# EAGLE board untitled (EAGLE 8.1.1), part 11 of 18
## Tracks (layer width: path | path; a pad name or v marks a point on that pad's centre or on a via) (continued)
S$10909 (continued)
  Bottom 0: 84.24,134.12 84.26,134.19
S$10910
  Bottom 0: 84.26,134.19 84.28,134.25
S$10911
  Bottom 0: 84.28,134.25 84.28,134.32
S$10912
  Bottom 0: 84.28,134.32 84.28,148.03
S$10913
  Bottom 0: 84.28,148.03 84.28,148.11
S$10914
  Bottom 0: 84.28,148.11 84.26,148.17
S$10915
  Bottom 0: 84.26,148.17 84.24,148.23
S$10916
  Bottom 0: 84.24,148.23 84.2,148.29
S$10917
  Bottom 0: 84.2,148.29 84.16,148.35
S$10918
  Bottom 0: 84.16,148.35 75.22,157.29
S$10919
  Bottom 0: 75.22,157.29 75.16,157.33
S$10920
  Bottom 0: 75.16,157.33 75.1,157.37
S$10921
  Bottom 0: 75.1,157.37 75.04,157.39
S$10922
  Bottom 0: 75.04,157.39 74.97,157.41
S$10923
  Bottom 0: 74.97,157.41 74.9,157.41
S$10924
  Bottom 0: 74.9,157.41 63.82,157.41
S$10925
  Bottom 0: 63.82,157.41 64.06,157.65
S$10926
  Bottom 0: 64.06,157.65 64.16,157.61
S$10927
  Bottom 0: 64.16,157.61 64.46,157.59
S$10928
  Bottom 0: 64.46,157.59 64.76,157.66
S$10929
  Bottom 0: 64.76,157.66 65.02,157.81
S$10930
  Bottom 0: 65.02,157.81 65.22,158.03
S$10931
  Bottom 0: 65.22,158.03 65.36,158.3
S$10932
  Bottom 0: 65.36,158.3 65.41,158.6
S$10933
  Bottom 0: 65.41,158.6 65.36,158.9
S$10934
  Bottom 0: 65.36,158.9 65.22,159.18
S$10935
  Bottom 0: 65.22,159.18 65.02,159.4
S$10936
  Bottom 0: 65.02,159.4 64.76,159.55
S$10937
  Bottom 0: 64.76,159.55 64.46,159.61
S$10938
  Bottom 0: 64.46,159.61 64.16,159.59
S$10939
  Bottom 0: 64.16,159.59 63.88,159.48
S$10940
  Bottom 0: 63.88,159.48 63.64,159.29
S$10941
  Bottom 0: 63.64,159.29 63.47,159.04
S$10942
  Bottom 0: 63.47,159.04 63.38,158.75
S$10943
  Bottom 0: 63.38,158.75 63.38,158.45
S$10944
  Bottom 0: 63.38,158.45 63.44,158.28
S$10945
  Bottom 0: 63.44,158.28 63.34,158.18
S$10946
  Bottom 0: 63.34,158.18 59.58,158.18
S$10947
  Bottom 0: 59.58,158.18 67.09,165.69
S$10948
  Bottom 0: 67.09,165.69 67.02,165.43
S$10949
  Bottom 0: 67.02,165.43 67.02,165.11
S$10950
  Bottom 0: 67.02,165.11 67.11,164.79
S$10951
  Bottom 0: 67.11,164.79 67.28,164.52
S$10952
  Bottom 0: 67.28,164.52 67.51,164.3
S$10953
  Bottom 0: 67.51,164.3 67.8,164.15
S$10954
  Bottom 0: 67.8,164.15 68.12,164.08
S$10955
  Bottom 0: 68.12,164.08 68.45,164.1
S$10956
  Bottom 0: 68.45,164.1 68.75,164.21
S$10957
  Bottom 0: 68.75,164.21 69.02,164.4
S$10958
  Bottom 0: 69.02,164.4 69.22,164.65
S$10959
  Bottom 0: 69.22,164.65 69.35,164.95
S$10960
  Bottom 0: 69.35,164.95 69.37,165.07
S$10961
  Bottom 0: 69.37,165.07 73.78,165.07
S$10962
  Bottom 0: 73.78,165.07 73.69,164.84
S$10963
  Bottom 0: 73.69,164.84 73.69,164.58
S$10964
  Bottom 0: 73.69,164.58 73.78,164.35
S$10965
  Bottom 0: 73.78,164.35 73.92,164.2
S$10966
  Bottom 0: 73.92,164.2 73.92,162.77
S$10967
  Bottom 0: 73.92,162.77 73.92,162.7
S$10968
  Bottom 0: 73.92,162.7 73.94,162.63
S$10969
  Bottom 0: 73.94,162.63 73.97,162.57
S$10970
  Bottom 0: 73.97,162.57 74,162.51
S$10971
  Bottom 0: 74,162.51 74.05,162.46
S$10972
  Bottom 0: 74.05,162.46 84.67,151.83
S$10973
  Bottom 0: 84.67,151.83 84.67,131.08
S$10974
  Bottom 0: 84.67,131.08 76.56,122.97
S$10975
  Bottom 0: 76.56,122.97 76.52,122.92
S$10976
  Bottom 0: 76.52,122.92 76.48,122.86
S$10977
  Bottom 0: 76.48,122.86 76.45,122.8
S$10978
  Bottom 0: 76.45,122.8 76.44,122.73
S$10979
  Bottom 0: 76.44,122.73 76.43,122.66
S$10980
  Bottom 0: 76.43,122.66 76.43,116.28
S$10981
  Bottom 0: 76.43,116.28 76.42,116.3
S$10982
  Bottom 0: 76.42,116.3 76.38,116.38
S$10983
  Bottom 0: 76.38,116.38 76.32,116.44
S$10984
  Bottom 0: 76.32,116.44 71.52,121.24
S$10985
  Bottom 0: 71.52,121.24 71.56,121.54
S$10986
  Bottom 0: 71.56,121.54 71.51,121.86
S$10987
  Bottom 0: 71.51,121.86 71.38,122.16
S$10988
  Bottom 0: 71.38,122.16 71.16,122.4
S$10989
  Bottom 0: 71.16,122.4 70.89,122.58
S$10990
  Bottom 0: 70.89,122.58 70.58,122.67
S$10991
  Bottom 0: 70.58,122.67 70.26,122.67
S$10992
  Bottom 0: 70.26,122.67 69.95,122.58
S$10993
  Bottom 0: 69.95,122.58 69.67,122.4
S$10994
  Bottom 0: 69.67,122.4 69.58,122.3
S$10995
  Bottom 0: 69.58,122.3 69.58,122.88
S$10996
  Bottom 0: 69.58,122.88 69.57,122.95
S$10997
  Bottom 0: 69.57,122.95 69.56,123.02
S$10998
  Bottom 0: 69.56,123.02 69.53,123.08
S$10999
  Bottom 0: 69.53,123.08 69.49,123.14
S$11000
  Bottom 0: 69.49,123.14 69.45,123.19
S$11001
  Bottom 0: 69.45,123.19 65.97,126.68
S$11002
  Bottom 0: 65.97,126.68 65.91,126.72
S$11003
  Bottom 0: 65.91,126.72 65.85,126.76
S$11004
  Bottom 0: 65.85,126.76 65.79,126.79
S$11005
  Bottom 0: 65.79,126.79 65.72,126.8
S$11006
  Bottom 0: 65.72,126.8 65.65,126.81
S$11007
  Bottom 0: 65.65,126.81 51.18,126.81
S$11008
  Bottom 0: 51.18,126.81 45.63,132.35
S$11009
  Bottom 0: 45.63,132.35 45.73,132.62
S$11010
  Bottom 0: 45.73,132.62 45.78,132.97
S$11011
  Bottom 0: 45.78,132.97 45.73,133.31
S$11012
  Bottom 0: 45.73,133.31 45.61,133.64
S$11013
  Bottom 0: 45.61,133.64 45.4,133.92
S$11014
  Bottom 0: 45.4,133.92 45.13,134.15
S$11015
  Bottom 0: 45.13,134.15 44.82,134.3
S$11016
  Bottom 0: 44.82,134.3 44.47,134.36
S$11017
  Bottom 0: 44.47,134.36 44.12,134.34
S$11018
  Bottom 0: 44.12,134.34 43.79,134.23
S$11019
  Bottom 0: 43.79,134.23 43.49,134.05
S$11020
  Bottom 0: 43.49,134.05 43.25,133.79
S$11021
  Bottom 0: 43.25,133.79 43.08,133.48
S$11022
  Bottom 0: 43.08,133.48 42.99,133.14
S$11023
  Bottom 0: 42.99,133.14 42.99,132.79
S$11024
  Bottom 0: 42.99,132.79 43.08,132.46
S$11025
  Bottom 0: 43.08,132.46 43.25,132.15
S$11026
  Bottom 0: 43.25,132.15 43.49,131.89
S$11027
  Bottom 0: 43.49,131.89 43.79,131.7
S$11028
  Bottom 0: 43.79,131.7 44.12,131.6
S$11029
  Bottom 0: 44.12,131.6 44.47,131.58
S$11030
  Bottom 0: 44.47,131.58 44.82,131.64
S$11031
  Bottom 0: 44.82,131.64 45,131.73
S$11032
  Bottom 0: 45,131.73 50.68,126.05
S$11033
  Bottom 0: 50.68,126.05 50.73,126.01
S$11034
  Bottom 0: 50.73,126.01 50.8,125.97
S$11035
  Bottom 0: 50.8,125.97 50.86,125.94
S$11036
  Bottom 0: 50.86,125.94 50.92,125.93
S$11037
  Bottom 0: 50.92,125.93 50.99,125.92
S$11038
  Bottom 0: 50.99,125.92 53.56,125.92
S$11039
  Bottom 0: 53.56,125.92 53.51,125.91
S$11040
  Bottom 0: 53.51,125.91 53.22,125.77
S$11041
  Bottom 0: 53.22,125.77 52.99,125.54
S$11042
  Bottom 0: 52.99,125.54 52.82,125.27
S$11043
  Bottom 0: 52.82,125.27 52.73,124.95
S$11044
  Bottom 0: 52.73,124.95 52.73,124.63
S$11045
  Bottom 0: 52.73,124.63 52.82,124.31
S$11046
  Bottom 0: 52.82,124.31 52.99,124.04
S$11047
  Bottom 0: 52.99,124.04 53.22,123.81
S$11048
  Bottom 0: 53.22,123.81 53.51,123.67
S$11049
  Bottom 0: 53.51,123.67 53.83,123.6
S$11050
  Bottom 0: 53.83,123.6 54.16,123.62
S$11051
  Bottom 0: 54.16,123.62 54.25,123.65
S$11052
  Bottom 0: 54.25,123.65 57.6,120.3
S$11053
  Bottom 0: 57.6,120.3 57.6,108.63
S$11054
  Bottom 0: 57.6,108.63 57.6,108.54
S$11055
  Bottom 0: 57.6,108.54 57.63,108.45
S$11056
  Bottom 0: 57.63,108.45 57.66,108.37
S$11057
  Bottom 0: 57.66,108.37 57.71,108.3
S$11058
  Bottom 0: 57.71,108.3 57.77,108.23
S$11059
  Bottom 0: 57.77,108.23 59.92,106.08
S$11060
  Bottom 0: 59.92,106.08 59.88,105.9
S$11061
  Bottom 0: 59.88,105.9 59.88,105.58
S$11062
  Bottom 0: 59.88,105.58 59.96,105.26
S$11063
  Bottom 0: 59.96,105.26 60.14,104.99
S$11064
  Bottom 0: 60.14,104.99 60.37,104.77
S$11065
  Bottom 0: 60.37,104.77 60.49,104.7
S$11066
  Bottom 0: 60.49,104.7 60.49,103.2
S$11067
  Bottom 0: 60.49,103.2 59.64,102.36
S$11068
  Bottom 0: 47.94,120.4 49.72,120.4
S$11069
  Bottom 0: 49.72,120.4 49.79,120.41
S$11070
  Bottom 0: 49.79,120.41 49.87,120.45
S$11071
  Bottom 0: 49.87,120.45 49.92,120.5
S$11072
  Bottom 0: 49.92,120.5 49.96,120.57
S$11073
  Bottom 0: 49.96,120.57 49.97,120.65
S$11074
  Bottom 0: 49.97,120.65 49.97,122.43
S$11075
  Bottom 0: 49.97,122.43 49.96,122.5
S$11076
  Bottom 0: 49.96,122.5 49.92,122.58
S$11077
  Bottom 0: 49.92,122.58 49.87,122.63
S$11078
  Bottom 0: 49.87,122.63 49.79,122.67
S$11079
  Bottom 0: 49.79,122.67 49.72,122.68
S$11080
  Bottom 0: 49.72,122.68 49.27,122.68
S$11081
  Bottom 0: 49.27,122.68 49.27,122.81
S$11082
  Bottom 0: 49.27,122.81 49.21,123.03
S$11083
  Bottom 0: 49.21,123.03 49.05,123.19
S$11084
  Bottom 0: 49.05,123.19 48.83,123.25
S$11085
  Bottom 0: 48.83,123.25 48.46,123.25
S$11086
  Bottom 0: 48.46,123.25 47.38,124.33
S$11087
  Bottom 0: 47.38,124.33 47.44,124.47
S$11088
  Bottom 0: 47.44,124.47 47.49,124.79
S$11089
  Bottom 0: 47.49,124.79 47.44,125.11
S$11090
  Bottom 0: 47.44,125.11 47.31,125.41
S$11091
  Bottom 0: 47.31,125.41 47.11,125.66
S$11092
  Bottom 0: 47.11,125.66 46.84,125.85
S$11093
  Bottom 0: 46.84,125.85 46.54,125.96
S$11094
  Bottom 0: 46.54,125.96 46.21,125.98
S$11095
  Bottom 0: 46.21,125.98 45.89,125.91
S$11096
  Bottom 0: 45.89,125.91 45.6,125.77
S$11097
  Bottom 0: 45.6,125.77 45.37,125.54
S$11098
  Bottom 0: 45.37,125.54 45.2,125.27
S$11099
  Bottom 0: 45.2,125.27 45.11,124.95
S$11100
  Bottom 0: 45.11,124.95 45.11,124.63
S$11101
  Bottom 0: 45.11,124.63 45.2,124.31
S$11102
  Bottom 0: 45.2,124.31 45.37,124.04
S$11103
  Bottom 0: 45.37,124.04 45.6,123.81
S$11104
  Bottom 0: 45.6,123.81 45.89,123.67
S$11105
  Bottom 0: 45.89,123.67 46.21,123.6
S$11106
  Bottom 0: 46.21,123.6 46.54,123.62
S$11107
  Bottom 0: 46.54,123.62 46.76,123.7
S$11108
  Bottom 0: 46.76,123.7 47.81,122.64
S$11109
  Bottom 0: 47.81,122.64 47.79,122.63
S$11110
  Bottom 0: 47.79,122.63 47.74,122.58
S$11111
  Bottom 0: 47.74,122.58 47.69,122.5
S$11112
  Bottom 0: 47.69,122.5 47.69,122.43
S$11113
  Bottom 0: 47.69,122.43 47.69,120.65
S$11114
  Bottom 0: 47.69,120.65 47.69,120.57
S$11115
  Bottom 0: 47.69,120.57 47.74,120.5
S$11116
  Bottom 0: 47.74,120.5 47.79,120.45
S$11117
  Bottom 0: 47.79,120.45 47.86,120.41
S$11118
  Bottom 0: 47.86,120.41 47.94,120.4
S$11119
  Bottom 0: 57.17,129.04 57.52,129.1
S$11120
  Bottom 0: 57.52,129.1 57.84,129.25
S$11121
  Bottom 0: 57.84,129.25 58.1,129.47
S$11122
  Bottom 0: 58.1,129.47 58.31,129.76
S$11123
  Bottom 0: 58.31,129.76 58.44,130.08
S$11124
  Bottom 0: 58.44,130.08 58.49,130.43
S$11125
  Bottom 0: 58.49,130.43 58.44,130.77
S$11126
  Bottom 0: 58.44,130.77 58.31,131.1
S$11127
  Bottom 0: 58.31,131.1 58.1,131.38
S$11128
  Bottom 0: 58.1,131.38 57.84,131.61
S$11129
  Bottom 0: 57.84,131.61 57.52,131.76
S$11130
  Bottom 0: 57.52,131.76 57.17,131.82
S$11131
  Bottom 0: 57.17,131.82 56.83,131.8
S$11132
  Bottom 0: 56.83,131.8 56.49,131.69
S$11133
  Bottom 0: 56.49,131.69 56.46,131.67
S$11134
  Bottom 0: 56.46,131.67 55.89,132.25
S$11135
  Bottom 0: 55.89,132.25 55.84,132.29
S$11136
  Bottom 0: 55.84,132.29 55.78,132.33
S$11137
  Bottom 0: 55.78,132.33 55.72,132.35
S$11138
  Bottom 0: 55.72,132.35 55.65,132.37
S$11139
  Bottom 0: 55.65,132.37 55.58,132.38
S$11140
  Bottom 0: 55.58,132.38 51.01,132.38
S$11141
  Bottom 0: 51.01,132.38 50.94,132.51
S$11142
  Bottom 0: 50.94,132.51 50.74,132.72
S$11143
  Bottom 0: 50.74,132.72 50.48,132.88
S$11144
  Bottom 0: 50.48,132.88 50.18,132.94
S$11145
  Bottom 0: 50.18,132.94 49.88,132.92
S$11146
  Bottom 0: 49.88,132.92 49.6,132.81
S$11147
  Bottom 0: 49.6,132.81 49.36,132.62
S$11148
  Bottom 0: 49.36,132.62 49.19,132.38
S$11149
  Bottom 0: 49.19,132.38 49.1,132.09
S$11150
  Bottom 0: 49.1,132.09 49.1,131.78
S$11151
  Bottom 0: 49.1,131.78 49.19,131.49
S$11152
  Bottom 0: 49.19,131.49 49.36,131.24
S$11153
  Bottom 0: 49.36,131.24 49.6,131.05
S$11154
  Bottom 0: 49.6,131.05 49.88,130.94
S$11155
  Bottom 0: 49.88,130.94 50.18,130.92
S$11156
  Bottom 0: 50.18,130.92 50.48,130.99
S$11157
  Bottom 0: 50.48,130.99 50.74,131.14
S$11158
  Bottom 0: 50.74,131.14 50.94,131.36
S$11159
  Bottom 0: 50.94,131.36 51.01,131.49
S$11160
  Bottom 0: 51.01,131.49 55.4,131.49
S$11161
  Bottom 0: 55.4,131.49 55.84,131.04
S$11162
  Bottom 0: 55.84,131.04 55.79,130.94
S$11163
  Bottom 0: 55.79,130.94 55.7,130.6
S$11164
  Bottom 0: 55.7,130.6 55.7,130.25
S$11165
  Bottom 0: 55.7,130.25 55.79,129.92
S$11166
  Bottom 0: 55.79,129.92 55.96,129.61
S$11167
  Bottom 0: 55.96,129.61 56.2,129.35
S$11168
  Bottom 0: 56.2,129.35 56.49,129.16
S$11169
  Bottom 0: 56.49,129.16 56.83,129.06
S$11170
  Bottom 0: 56.83,129.06 57.17,129.04
S$11171
  Bottom 0: 83.52,149.97 83.81,150.04
S$11172
  Bottom 0: 83.81,150.04 84.08,150.19
S$11173
  Bottom 0: 84.08,150.19 84.28,150.41
S$11174
  Bottom 0: 84.28,150.41 84.41,150.68
S$11175
  Bottom 0: 84.41,150.68 84.46,150.98
S$11176
  Bottom 0: 84.46,150.98 84.41,151.28
S$11177
  Bottom 0: 84.41,151.28 84.28,151.56
S$11178
  Bottom 0: 84.28,151.56 84.08,151.78
S$11179
  Bottom 0: 84.08,151.78 83.81,151.93
S$11180
  Bottom 0: 83.81,151.93 83.52,151.99
S$11181
  Bottom 0: 83.52,151.99 83.22,151.97
S$11182
  Bottom 0: 83.22,151.97 82.94,151.86
S$11183
  Bottom 0: 82.94,151.86 82.7,151.67
S$11184
  Bottom 0: 82.7,151.67 82.53,151.43
S$11185
  Bottom 0: 82.53,151.43 82.44,151.13
S$11186
  Bottom 0: 82.44,151.13 82.44,150.83
S$11187
  Bottom 0: 82.44,150.83 82.53,150.54
S$11188
  Bottom 0: 82.53,150.54 82.7,150.29
S$11189
  Bottom 0: 82.7,150.29 82.94,150.1
S$11190
  Bottom 0: 82.94,150.1 83.22,149.99
S$11191
  Bottom 0: 83.22,149.99 83.52,149.97
S$11192
  Bottom 0: 71.75,158.5 73.53,158.5
S$11193
  Bottom 0: 73.53,158.5 73.61,158.51
S$11194
  Bottom 0: 73.61,158.51 73.68,158.55
S$11195
  Bottom 0: 73.68,158.55 73.73,158.6
S$11196
  Bottom 0: 73.73,158.6 73.78,158.67
S$11197
  Bottom 0: 73.78,158.67 73.79,158.75
S$11198
  Bottom 0: 73.79,158.75 73.79,160.53
S$11199
  Bottom 0: 73.79,160.53 73.78,160.6
S$11200
  Bottom 0: 73.78,160.6 73.73,160.68
S$11201
  Bottom 0: 73.73,160.68 73.68,160.73
S$11202
  Bottom 0: 73.68,160.73 73.61,160.77
S$11203
  Bottom 0: 73.61,160.77 73.53,160.78
S$11204
  Bottom 0: 73.53,160.78 73.09,160.78
S$11205
  Bottom 0: 73.09,160.78 73.09,160.91
S$11206
  Bottom 0: 73.09,160.91 73.03,161.13
S$11207
  Bottom 0: 73.03,161.13 72.86,161.29
S$11208
  Bottom 0: 72.86,161.29 72.64,161.35
S$11209
  Bottom 0: 72.64,161.35 72.28,161.35
S$11210
  Bottom 0: 72.28,161.35 71.19,162.43
S$11211
  Bottom 0: 71.19,162.43 71.25,162.57
S$11212
  Bottom 0: 71.25,162.57 71.3,162.89
S$11213
  Bottom 0: 71.3,162.89 71.25,163.22
S$11214
  Bottom 0: 71.25,163.22 71.13,163.51
S$11215
  Bottom 0: 71.13,163.51 70.92,163.77
S$11216
  Bottom 0: 70.92,163.77 70.66,163.96
S$11217
  Bottom 0: 70.66,163.96 70.35,164.06
S$11218
  Bottom 0: 70.35,164.06 70.03,164.08
S$11219
  Bottom 0: 70.03,164.08 69.71,164.02
S$11220
  Bottom 0: 69.71,164.02 69.42,163.87
S$11221
  Bottom 0: 69.42,163.87 69.19,163.65
S$11222
  Bottom 0: 69.19,163.65 69.01,163.37
S$11223
  Bottom 0: 69.01,163.37 68.92,163.06
S$11224
  Bottom 0: 68.92,163.06 68.92,162.73
S$11225
  Bottom 0: 68.92,162.73 69.01,162.42
S$11226
  Bottom 0: 69.01,162.42 69.19,162.14
S$11227
  Bottom 0: 69.19,162.14 69.42,161.92
S$11228
  Bottom 0: 69.42,161.92 69.71,161.77
S$11229
  Bottom 0: 69.71,161.77 70.03,161.71
S$11230
  Bottom 0: 70.03,161.71 70.35,161.73
S$11231
  Bottom 0: 70.35,161.73 70.58,161.8
S$11232
  Bottom 0: 70.58,161.8 71.64,160.75
S$11233
  Bottom 0: 71.64,160.75 71.61,160.73
S$11234
  Bottom 0: 71.61,160.73 71.55,160.68
S$11235
  Bottom 0: 71.55,160.68 71.51,160.6
S$11236
  Bottom 0: 71.51,160.6 71.5,160.53
S$11237
  Bottom 0: 71.5,160.53 71.5,158.75
S$11238
  Bottom 0: 71.5,158.75 71.51,158.67
S$11239
  Bottom 0: 71.51,158.67 71.55,158.6
S$11240
  Bottom 0: 71.55,158.6 71.61,158.55
S$11241
  Bottom 0: 71.61,158.55 71.68,158.51
S$11242
  Bottom 0: 71.68,158.51 71.75,158.5
S$11243
  Bottom 0: 75.02,158.51 75.35,158.51
S$11244
  Bottom 0: 75.35,158.51 75.66,158.6
S$11245
  Bottom 0: 75.66,158.6 75.93,158.78
S$11246
  Bottom 0: 75.93,158.78 76.14,159.02
S$11247
  Bottom 0: 76.14,159.02 76.28,159.32
S$11248
  Bottom 0: 76.28,159.32 76.33,159.64
S$11249
  Bottom 0: 76.33,159.64 76.28,159.96
S$11250
  Bottom 0: 76.28,159.96 76.14,160.26
S$11251
  Bottom 0: 76.14,160.26 75.93,160.5
S$11252
  Bottom 0: 75.93,160.5 75.66,160.68
S$11253
  Bottom 0: 75.66,160.68 75.35,160.77
S$11254
  Bottom 0: 75.35,160.77 75.02,160.77
S$11255
  Bottom 0: 75.02,160.77 74.71,160.68
S$11256
  Bottom 0: 74.71,160.68 74.44,160.5
S$11257
  Bottom 0: 74.44,160.5 74.22,160.26
S$11258
  Bottom 0: 74.22,160.26 74.08,159.96
S$11259
  Bottom 0: 74.08,159.96 74.04,159.64
S$11260
  Bottom 0: 74.04,159.64 74.08,159.32
S$11261
  Bottom 0: 74.08,159.32 74.22,159.02
S$11262
  Bottom 0: 74.22,159.02 74.44,158.78
S$11263
  Bottom 0: 74.44,158.78 74.71,158.6
S$11264
  Bottom 0: 74.71,158.6 75.02,158.51
S$11265
  Bottom 0: 226.34,102.45 226.34,102.49
S$11266
  Bottom 0: 226.34,102.49 226.3,102.81
S$11267
  Bottom 0: 226.3,102.81 226.16,103.11
S$11268
  Bottom 0: 226.16,103.11 225.95,103.35
S$11269
  Bottom 0: 225.95,103.35 225.67,103.53
S$11270
  Bottom 0: 225.67,103.53 225.36,103.62
S$11271
  Bottom 0: 225.36,103.62 225.25,103.62
S$11272
  Bottom 0: 225.25,103.62 219.09,109.79
S$11273
  Bottom 0: 219.09,109.79 219.02,109.85
S$11274
  Bottom 0: 219.02,109.85 218.94,109.9
S$11275
  Bottom 0: 218.94,109.9 218.86,109.93
S$11276
  Bottom 0: 218.86,109.93 218.78,109.95
S$11277
  Bottom 0: 218.78,109.95 218.68,109.96
S$11278
  Bottom 0: 218.68,109.96 218.59,109.96
S$11279
  Bottom 0: 218.59,109.96 218.44,110.1
S$11280
  Bottom 0: 218.44,110.1 218.75,110.01
S$11281
  Bottom 0: 218.75,110.01 219.09,109.99
S$11282
  Bottom 0: 219.09,109.99 219.44,110.05
S$11283
  Bottom 0: 219.44,110.05 219.76,110.2
S$11284
  Bottom 0: 219.76,110.2 220.03,110.42
S$11285
  Bottom 0: 220.03,110.42 220.23,110.71
S$11286
  Bottom 0: 220.23,110.71 220.36,111.03
S$11287
  Bottom 0: 220.36,111.03 220.41,111.38
S$11288
  Bottom 0: 220.41,111.38 220.36,111.72
S$11289
  Bottom 0: 220.36,111.72 220.23,112.05
S$11290
  Bottom 0: 220.23,112.05 220.03,112.33
S$11291
  Bottom 0: 220.03,112.33 219.76,112.56
S$11292
  Bottom 0: 219.76,112.56 219.44,112.71
S$11293
  Bottom 0: 219.44,112.71 219.09,112.77
S$11294
  Bottom 0: 219.09,112.77 218.75,112.75
S$11295
  Bottom 0: 218.75,112.75 218.41,112.64
S$11296
  Bottom 0: 218.41,112.64 218.12,112.46
S$11297
  Bottom 0: 218.12,112.46 217.91,112.23
S$11298
  Bottom 0: 217.91,112.23 217.91,115.83
S$11299
  Bottom 0: 217.91,115.83 219.46,117.38
S$11300
  Bottom 0: 219.46,117.38 219.44,117.33
S$11301
  Bottom 0: 219.44,117.33 219.31,116.91
S$11302
  Bottom 0: 219.31,116.91 219.26,116.46
S$11303
  Bottom 0: 219.26,116.46 219.31,116.01
S$11304
  Bottom 0: 219.31,116.01 219.44,115.58
S$11305
  Bottom 0: 219.44,115.58 219.65,115.19
S$11306
  Bottom 0: 219.65,115.19 219.93,114.84
S$11307
  Bottom 0: 219.93,114.84 220.28,114.56
S$11308
  Bottom 0: 220.28,114.56 220.68,114.35
S$11309
  Bottom 0: 220.68,114.35 221.1,114.22
S$11310
  Bottom 0: 221.1,114.22 221.55,114.17
S$11311
  Bottom 0: 221.55,114.17 222,114.22
S$11312
  Bottom 0: 222,114.22 222.42,114.35
S$11313
  Bottom 0: 222.42,114.35 222.82,114.56
S$11314
  Bottom 0: 222.82,114.56 223.16,114.84
S$11315
  Bottom 0: 223.16,114.84 223.45,115.19
S$11316
  Bottom 0: 223.45,115.19 223.66,115.58
S$11317
  Bottom 0: 223.66,115.58 223.79,116.01
S$11318
  Bottom 0: 223.79,116.01 223.84,116.46
S$11319
  Bottom 0: 223.84,116.46 223.79,116.91
S$11320
  Bottom 0: 223.79,116.91 223.66,117.33
S$11321
  Bottom 0: 223.66,117.33 223.45,117.73
S$11322
  Bottom 0: 223.45,117.73 223.16,118.07
S$11323
  Bottom 0: 223.16,118.07 222.82,118.36
S$11324
  Bottom 0: 222.82,118.36 222.42,118.57
S$11325
  Bottom 0: 222.42,118.57 222,118.7
S$11326
  Bottom 0: 222,118.7 221.55,118.75
S$11327
  Bottom 0: 221.55,118.75 221.1,118.7
S$11328
  Bottom 0: 221.1,118.7 220.68,118.57
S$11329
  Bottom 0: 220.68,118.57 220.62,118.55
S$11330
  Bottom 0: 220.62,118.55 222.52,120.45
S$11331
  Bottom 0: 222.52,120.45 222.65,120.41
S$11332
  Bottom 0: 222.65,120.41 222.98,120.41
S$11333
  Bottom 0: 222.98,120.41 223.29,120.5
S$11334
  Bottom 0: 223.29,120.5 223.57,120.67
S$11335
  Bottom 0: 223.57,120.67 223.78,120.92
S$11336
  Bottom 0: 223.78,120.92 223.92,121.22
S$11337
  Bottom 0: 223.92,121.22 223.96,121.54
S$11338
  Bottom 0: 223.96,121.54 223.92,121.86
S$11339
  Bottom 0: 223.92,121.86 223.78,122.16
S$11340
  Bottom 0: 223.78,122.16 223.57,122.4
S$11341
  Bottom 0: 223.57,122.4 223.29,122.58
S$11342
  Bottom 0: 223.29,122.58 223.24,122.6
S$11343
  Bottom 0: 223.24,122.6 223.24,123.02
S$11344
  Bottom 0: 223.24,123.02 223.25,123.01
S$11345
  Bottom 0: 223.25,123.01 223.29,122.96
S$11346
  Bottom 0: 223.29,122.96 224.92,121.33
S$11347
  Bottom 0: 224.92,121.33 224.92,115.23
S$11348
  Bottom 0: 224.92,115.23 224.76,115.18
S$11349
  Bottom 0: 224.76,115.18 224.47,115
S$11350
  Bottom 0: 224.47,115 224.23,114.74
S$11351
  Bottom 0: 224.23,114.74 224.06,114.43
S$11352
  Bottom 0: 224.06,114.43 223.97,114.09
S$11353
  Bottom 0: 223.97,114.09 223.97,113.75
S$11354
  Bottom 0: 223.97,113.75 224.06,113.41
S$11355
  Bottom 0: 224.06,113.41 224.23,113.1
S$11356
  Bottom 0: 224.23,113.1 224.47,112.84
S$11357
  Bottom 0: 224.47,112.84 224.76,112.65
S$11358
  Bottom 0: 224.76,112.65 225.09,112.55
S$11359
  Bottom 0: 225.09,112.55 225.44,112.53
S$11360
  Bottom 0: 225.44,112.53 225.79,112.59
S$11361
  Bottom 0: 225.79,112.59 226.11,112.74
S$11362
  Bottom 0: 226.11,112.74 226.38,112.96
S$11363
  Bottom 0: 226.38,112.96 226.58,113.25
S$11364
  Bottom 0: 226.58,113.25 226.71,113.57
S$11365
  Bottom 0: 226.71,113.57 226.76,113.92
S$11366
  Bottom 0: 226.76,113.92 226.71,114.26
S$11367
  Bottom 0: 226.71,114.26 226.58,114.59
S$11368
  Bottom 0: 226.58,114.59 226.38,114.87
S$11369
  Bottom 0: 226.38,114.87 226.11,115.1
S$11370
  Bottom 0: 226.11,115.1 225.8,115.25
S$11371
  Bottom 0: 225.8,115.25 225.8,121.51
S$11372
  Bottom 0: 225.8,121.51 225.8,121.58
S$11373
  Bottom 0: 225.8,121.58 225.78,121.65
S$11374
  Bottom 0: 225.78,121.65 225.75,121.71
S$11375
  Bottom 0: 225.75,121.71 225.72,121.77
S$11376
  Bottom 0: 225.72,121.77 225.67,121.83
S$11377
  Bottom 0: 225.67,121.83 224.04,123.46
S$11378
  Bottom 0: 224.04,123.46 224.04,126.22
S$11379
  Bottom 0: 224.04,126.22 224.11,126.27
S$11380
  Bottom 0: 224.11,126.27 224.24,126.48
S$11381
  Bottom 0: 224.24,126.48 224.29,126.73
S$11382
  Bottom 0: 224.29,126.73 224.24,126.98
S$11383
  Bottom 0: 224.24,126.98 224.11,127.19
S$11384
  Bottom 0: 224.11,127.19 223.91,127.34
S$11385
  Bottom 0: 223.91,127.34 223.66,127.41
S$11386
  Bottom 0: 223.66,127.41 223.41,127.39
S$11387
  Bottom 0: 223.41,127.39 223.24,127.31
S$11388
  Bottom 0: 223.24,127.31 223.24,128.66
S$11389
  Bottom 0: 223.24,128.66 223.24,128.75
S$11390
  Bottom 0: 223.24,128.75 223.22,128.83
S$11391
  Bottom 0: 223.22,128.83 223.18,128.91
S$11392
  Bottom 0: 223.18,128.91 223.13,128.99
S$11393
  Bottom 0: 223.13,128.99 223.07,129.06
S$11394
  Bottom 0: 223.07,129.06 221.09,131.04
S$11395
  Bottom 0: 221.09,131.04 221.34,130.94
S$11396
  Bottom 0: 221.34,130.94 221.64,130.92
S$11397
  Bottom 0: 221.64,130.92 221.89,130.98
S$11398
  Bottom 0: 221.89,130.98 222.76,130.11
S$11399
  Bottom 0: 222.76,130.11 222.81,130.07
S$11400
  Bottom 0: 222.81,130.07 222.88,130.03
S$11401
  Bottom 0: 222.88,130.03 222.94,130.01
S$11402
  Bottom 0: 222.94,130.01 223,129.99
S$11403
  Bottom 0: 223,129.99 223.07,129.99
S$11404
  Bottom 0: 223.07,129.99 227.21,129.99
S$11405
  Bottom 0: 227.21,129.99 227.23,129.92
S$11406
  Bottom 0: 227.23,129.92 227.41,129.61
S$11407
  Bottom 0: 227.41,129.61 227.65,129.35
S$11408
  Bottom 0: 227.65,129.35 227.94,129.16
S$11409
  Bottom 0: 227.94,129.16 228.27,129.06
S$11410
  Bottom 0: 228.27,129.06 228.62,129.04
S$11411
  Bottom 0: 228.62,129.04 228.97,129.1
S$11412
  Bottom 0: 228.97,129.1 229.28,129.25
S$11413
  Bottom 0: 229.28,129.25 229.55,129.47
S$11414
  Bottom 0: 229.55,129.47 229.76,129.76
S$11415
  Bottom 0: 229.76,129.76 229.88,130.08
S$11416
  Bottom 0: 229.88,130.08 229.93,130.43
S$11417
  Bottom 0: 229.93,130.43 229.88,130.77
S$11418
  Bottom 0: 229.88,130.77 229.76,131.1
S$11419
  Bottom 0: 229.76,131.1 229.55,131.38
S$11420
  Bottom 0: 229.55,131.38 229.28,131.61
S$11421
  Bottom 0: 229.28,131.61 228.97,131.76
S$11422
  Bottom 0: 228.97,131.76 228.62,131.82
S$11423
  Bottom 0: 228.62,131.82 228.27,131.8
S$11424
  Bottom 0: 228.27,131.8 227.94,131.69
S$11425
  Bottom 0: 227.94,131.69 227.65,131.51
S$11426
  Bottom 0: 227.65,131.51 227.41,131.25
S$11427
  Bottom 0: 227.41,131.25 227.23,130.94
S$11428
  Bottom 0: 227.23,130.94 227.21,130.87
S$11429
  Bottom 0: 227.21,130.87 223.26,130.87
S$11430
  Bottom 0: 223.26,130.87 222.52,131.61
S$11431
  Bottom 0: 222.52,131.61 222.54,131.63
S$11432
  Bottom 0: 222.54,131.63 222.59,131.93
S$11433
  Bottom 0: 222.59,131.93 222.54,132.23
S$11434
  Bottom 0: 222.54,132.23 222.41,132.51
S$11435
  Bottom 0: 222.41,132.51 222.2,132.72
S$11436
  Bottom 0: 222.2,132.72 221.94,132.88
S$11437
  Bottom 0: 221.94,132.88 221.64,132.94
S$11438
  Bottom 0: 221.64,132.94 221.34,132.92
S$11439
  Bottom 0: 221.34,132.92 221.06,132.81
S$11440
  Bottom 0: 221.06,132.81 220.82,132.62
S$11441
  Bottom 0: 220.82,132.62 220.66,132.38
S$11442
  Bottom 0: 220.66,132.38 220.56,132.09
S$11443
  Bottom 0: 220.56,132.09 220.56,131.78
S$11444
  Bottom 0: 220.56,131.78 220.66,131.49
S$11445
  Bottom 0: 220.66,131.49 220.68,131.44
S$11446
  Bottom 0: 220.68,131.44 217.47,134.66
S$11447
  Bottom 0: 217.47,134.66 217.47,136.98
S$11448
  Bottom 0: 217.47,136.98 217.47,137.07
S$11449
  Bottom 0: 217.47,137.07 217.45,137.16
S$11450
  Bottom 0: 217.45,137.16 217.41,137.23
S$11451
  Bottom 0: 217.41,137.23 217.37,137.31
S$11452
  Bottom 0: 217.37,137.31 217.31,137.38
S$11453
  Bottom 0: 217.31,137.38 214.4,140.29
S$11454
  Bottom 0: 214.4,140.29 214.44,140.59
S$11455
  Bottom 0: 214.44,140.59 214.39,140.91
S$11456
  Bottom 0: 214.39,140.91 214.25,141.21
S$11457
  Bottom 0: 214.25,141.21 214.04,141.45
S$11458
  Bottom 0: 214.04,141.45 213.76,141.63
S$11459
  Bottom 0: 213.76,141.63 213.46,141.72
S$11460
  Bottom 0: 213.46,141.72 213.13,141.72
S$11461
  Bottom 0: 213.13,141.72 212.82,141.63
S$11462
  Bottom 0: 212.82,141.63 212.55,141.45
S$11463
  Bottom 0: 212.55,141.45 212.33,141.21
S$11464
  Bottom 0: 212.33,141.21 212.2,140.91
S$11465
  Bottom 0: 212.2,140.91 212.15,140.59
S$11466
  Bottom 0: 212.15,140.59 212.2,140.27
S$11467
  Bottom 0: 212.2,140.27 212.33,139.97
S$11468
  Bottom 0: 212.33,139.97 212.55,139.72
S$11469
  Bottom 0: 212.55,139.72 212.82,139.55
S$11470
  Bottom 0: 212.82,139.55 213.13,139.46
S$11471
  Bottom 0: 213.13,139.46 213.46,139.46
S$11472
  Bottom 0: 213.46,139.46 213.58,139.5
S$11473
  Bottom 0: 213.58,139.5 216.34,136.74
S$11474
  Bottom 0: 216.34,136.74 216.34,134.42
S$11475
  Bottom 0: 216.34,134.42 216.34,134.33
S$11476
  Bottom 0: 216.34,134.33 216.36,134.25
S$11477
  Bottom 0: 216.36,134.25 216.28,134.29
S$11478
  Bottom 0: 216.28,134.29 216.28,135.1
S$11479
  Bottom 0: 216.28,135.1 216.27,135.17
S$11480
  Bottom 0: 216.27,135.17 216.26,135.24
S$11481
  Bottom 0: 216.26,135.24 216.23,135.3
S$11482
  Bottom 0: 216.23,135.3 216.19,135.36
S$11483
  Bottom 0: 216.19,135.36 216.15,135.41
S$11484
  Bottom 0: 216.15,135.41 213.34,138.23
S$11485
  Bottom 0: 213.34,138.23 213.28,138.27
S$11486
  Bottom 0: 213.28,138.27 213.22,138.31
S$11487
  Bottom 0: 213.22,138.31 213.16,138.33
S$11488
  Bottom 0: 213.16,138.33 213.09,138.35
S$11489
  Bottom 0: 213.09,138.35 213.02,138.35
S$11490
  Bottom 0: 213.02,138.35 206.21,138.35
S$11491
  Bottom 0: 206.21,138.35 197.36,147.2
S$11492
  Bottom 0: 197.36,147.2 197.3,147.24
S$11493
  Bottom 0: 197.3,147.24 197.24,147.28
S$11494
  Bottom 0: 197.24,147.28 197.18,147.31
S$11495
  Bottom 0: 197.18,147.31 197.11,147.32
S$11496
  Bottom 0: 197.11,147.32 197.04,147.32
S$11497
  Bottom 0: 197.04,147.32 178.29,147.32
S$11498
  Bottom 0: 178.29,147.32 174.22,151.4
S$11499
  Bottom 0: 174.22,151.4 174.32,151.67
S$11500
  Bottom 0: 174.32,151.67 174.37,152.02
S$11501
  Bottom 0: 174.37,152.02 174.32,152.36
S$11502
  Bottom 0: 174.32,152.36 174.2,152.69
S$11503
  Bottom 0: 174.2,152.69 173.99,152.97
S$11504
  Bottom 0: 173.99,152.97 173.81,153.12
S$11505
  Bottom 0: 173.81,153.12 175.39,153.12
S$11506
  Bottom 0: 175.39,153.12 176.67,151.84
S$11507
  Bottom 0: 176.67,151.84 176.72,151.81
S$11508
  Bottom 0: 176.72,151.81 176.78,151.76
S$11509
  Bottom 0: 176.78,151.76 176.84,151.74
S$11510
  Bottom 0: 176.84,151.74 176.91,151.72
S$11511
  Bottom 0: 176.91,151.72 176.98,151.72
S$11512
  Bottom 0: 176.98,151.72 178.01,151.72
S$11513
  Bottom 0: 178.01,151.72 177.96,151.67
S$11514
  Bottom 0: 177.96,151.67 177.79,151.43
S$11515
  Bottom 0: 177.79,151.43 177.7,151.13
S$11516
  Bottom 0: 177.7,151.13 177.7,150.83
S$11517
  Bottom 0: 177.7,150.83 177.79,150.54
S$11518
  Bottom 0: 177.79,150.54 177.96,150.29
S$11519
  Bottom 0: 177.96,150.29 178.2,150.1
S$11520
  Bottom 0: 178.2,150.1 178.48,149.99
S$11521
  Bottom 0: 178.48,149.99 178.78,149.97
S$11522
  Bottom 0: 178.78,149.97 179.07,150.04
S$11523
  Bottom 0: 179.07,150.04 179.34,150.19
S$11524
  Bottom 0: 179.34,150.19 179.54,150.41
S$11525
  Bottom 0: 179.54,150.41 179.61,150.54
S$11526
  Bottom 0: 179.61,150.54 183.98,150.54
S$11527
  Bottom 0: 183.98,150.54 184.43,150.09
S$11528
  Bottom 0: 184.43,150.09 184.37,149.99
S$11529
  Bottom 0: 184.37,149.99 184.29,149.65
S$11530
  Bottom 0: 184.29,149.65 184.29,149.3
S$11531
  Bottom 0: 184.29,149.3 184.37,148.97
S$11532
  Bottom 0: 184.37,148.97 184.55,148.66
S$11533
  Bottom 0: 184.55,148.66 184.78,148.4
S$11534
  Bottom 0: 184.78,148.4 185.08,148.21
S$11535
  Bottom 0: 185.08,148.21 185.41,148.11
S$11536
  Bottom 0: 185.41,148.11 185.76,148.09
S$11537
  Bottom 0: 185.76,148.09 186.11,148.15
S$11538
  Bottom 0: 186.11,148.15 186.42,148.3
S$11539
  Bottom 0: 186.42,148.3 186.69,148.52
S$11540
  Bottom 0: 186.69,148.52 186.9,148.81
S$11541
  Bottom 0: 186.9,148.81 187.03,149.13
S$11542
  Bottom 0: 187.03,149.13 187.07,149.48
S$11543
  Bottom 0: 187.07,149.48 187.03,149.82
S$11544
  Bottom 0: 187.03,149.82 186.9,150.15
S$11545
  Bottom 0: 186.9,150.15 186.69,150.43
S$11546
  Bottom 0: 186.69,150.43 186.42,150.66
S$11547
  Bottom 0: 186.42,150.66 186.11,150.81
S$11548
  Bottom 0: 186.11,150.81 185.76,150.87
S$11549
  Bottom 0: 185.76,150.87 185.41,150.85
S$11550
  Bottom 0: 185.41,150.85 185.08,150.74
S$11551
  Bottom 0: 185.08,150.74 185.05,150.73
S$11552
  Bottom 0: 185.05,150.73 184.49,151.3
S$11553
  Bottom 0: 184.49,151.3 184.43,151.34
S$11554
  Bottom 0: 184.43,151.34 184.37,151.38
S$11555
  Bottom 0: 184.37,151.38 184.31,151.4
S$11556
  Bottom 0: 184.31,151.4 184.24,151.42
S$11557
  Bottom 0: 184.24,151.42 184.17,151.43
S$11558
  Bottom 0: 184.17,151.43 179.61,151.43
S$11559
  Bottom 0: 179.61,151.43 179.54,151.56
S$11560
  Bottom 0: 179.54,151.56 179.39,151.72
S$11561
  Bottom 0: 179.39,151.72 190.67,151.72
S$11562
  Bottom 0: 190.67,151.72 190.72,151.51
S$11563
  Bottom 0: 190.72,151.51 190.9,151.2
S$11564
  Bottom 0: 190.9,151.2 191.13,150.94
S$11565
  Bottom 0: 191.13,150.94 191.43,150.75
S$11566
  Bottom 0: 191.43,150.75 191.76,150.65
S$11567
  Bottom 0: 191.76,150.65 192.11,150.63
S$11568
  Bottom 0: 192.11,150.63 192.46,150.69
S$11569
  Bottom 0: 192.46,150.69 192.77,150.84
S$11570
  Bottom 0: 192.77,150.84 193.04,151.06
S$11571
  Bottom 0: 193.04,151.06 193.25,151.35
S$11572
  Bottom 0: 193.25,151.35 193.38,151.67
S$11573
  Bottom 0: 193.38,151.67 193.42,152.02
S$11574
  Bottom 0: 193.42,152.02 193.38,152.36
S$11575
  Bottom 0: 193.38,152.36 193.25,152.69
S$11576
  Bottom 0: 193.25,152.69 193.04,152.97
S$11577
  Bottom 0: 193.04,152.97 192.77,153.2
S$11578
  Bottom 0: 192.77,153.2 192.47,153.34
S$11579
  Bottom 0: 192.47,153.34 192.47,154.51
S$11580
  Bottom 0: 192.47,154.51 196.76,158.81
S$11581
  Bottom 0: 196.76,158.81 196.75,158.75
S$11582
  Bottom 0: 196.75,158.75 196.75,158.45
S$11583
  Bottom 0: 196.75,158.45 196.84,158.16
S$11584
  Bottom 0: 196.84,158.16 197,157.91
S$11585
  Bottom 0: 197,157.91 197.25,157.72
S$11586
  Bottom 0: 197.25,157.72 197.53,157.61
S$11587
  Bottom 0: 197.53,157.61 197.83,157.59
S$11588
  Bottom 0: 197.83,157.59 198.08,157.65
S$11589
  Bottom 0: 198.08,157.65 204.87,150.86
S$11590
  Bottom 0: 204.87,150.86 204.81,150.87
S$11591
  Bottom 0: 204.81,150.87 204.46,150.85
S$11592
  Bottom 0: 204.46,150.85 204.13,150.74
S$11593
  Bottom 0: 204.13,150.74 204.1,150.72
S$11594
  Bottom 0: 204.1,150.72 203.53,151.3
S$11595
  Bottom 0: 203.53,151.3 203.47,151.34
S$11596
  Bottom 0: 203.47,151.34 203.41,151.38
S$11597
  Bottom 0: 203.41,151.38 203.35,151.4
S$11598
  Bottom 0: 203.35,151.4 203.28,151.42
S$11599
  Bottom 0: 203.28,151.42 203.22,151.43
S$11600
  Bottom 0: 203.22,151.43 198.66,151.43
S$11601
  Bottom 0: 198.66,151.43 198.59,151.56
S$11602
  Bottom 0: 198.59,151.56 198.39,151.78
S$11603
  Bottom 0: 198.39,151.78 198.12,151.93
S$11604
  Bottom 0: 198.12,151.93 197.83,151.99
S$11605
  Bottom 0: 197.83,151.99 197.53,151.97
S$11606
  Bottom 0: 197.53,151.97 197.25,151.86
S$11607
  Bottom 0: 197.25,151.86 197,151.67
S$11608
  Bottom 0: 197,151.67 196.84,151.43
S$11609
  Bottom 0: 196.84,151.43 196.75,151.13
S$11610
  Bottom 0: 196.75,151.13 196.75,150.83
S$11611
  Bottom 0: 196.75,150.83 196.84,150.54
S$11612
  Bottom 0: 196.84,150.54 197,150.29
S$11613
  Bottom 0: 197,150.29 197.25,150.1
S$11614
  Bottom 0: 197.25,150.1 197.53,149.99
S$11615
  Bottom 0: 197.53,149.99 197.83,149.97
S$11616
  Bottom 0: 197.83,149.97 198.12,150.04
S$11617
  Bottom 0: 198.12,150.04 198.39,150.19
S$11618
  Bottom 0: 198.39,150.19 198.59,150.41
S$11619
  Bottom 0: 198.59,150.41 198.66,150.54
S$11620
  Bottom 0: 198.66,150.54 203.03,150.54
S$11621
  Bottom 0: 203.03,150.54 203.48,150.09
S$11622
  Bottom 0: 203.48,150.09 203.42,149.99
S$11623
  Bottom 0: 203.42,149.99 203.34,149.65
S$11624
  Bottom 0: 203.34,149.65 203.34,149.3
S$11625
  Bottom 0: 203.34,149.3 203.42,148.97
S$11626
  Bottom 0: 203.42,148.97 203.6,148.66
S$11627
  Bottom 0: 203.6,148.66 203.84,148.4
S$11628
  Bottom 0: 203.84,148.4 204.13,148.21
S$11629
  Bottom 0: 204.13,148.21 204.46,148.11
S$11630
  Bottom 0: 204.46,148.11 204.81,148.09
S$11631
  Bottom 0: 204.81,148.09 205.16,148.15
S$11632
  Bottom 0: 205.16,148.15 205.47,148.3
S$11633
  Bottom 0: 205.47,148.3 205.74,148.52
S$11634
  Bottom 0: 205.74,148.52 205.95,148.81
S$11635
  Bottom 0: 205.95,148.81 206.07,149.13
S$11636
  Bottom 0: 206.07,149.13 206.12,149.48
S$11637
  Bottom 0: 206.12,149.48 206.1,149.63
S$11638
  Bottom 0: 206.1,149.63 223.63,132.09
S$11639
  Bottom 0: 223.63,132.09 223.69,132.06
S$11640
  Bottom 0: 223.69,132.06 223.75,132.01
S$11641
  Bottom 0: 223.75,132.01 223.81,131.99
S$11642
  Bottom 0: 223.81,131.99 223.88,131.97
S$11643
  Bottom 0: 223.88,131.97 223.95,131.97
S$11644
  Bottom 0: 223.95,131.97 232.4,131.97
S$11645
  Bottom 0: 232.4,131.97 233.22,131.14
S$11646
  Bottom 0: 233.22,131.14 233.28,131.1
S$11647
  Bottom 0: 233.28,131.1 233.34,131.06
S$11648
  Bottom 0: 233.34,131.06 233.4,131.04
S$11649
  Bottom 0: 233.4,131.04 233.47,131.02
S$11650
  Bottom 0: 233.47,131.02 233.54,131.02
S$11651
  Bottom 0: 233.54,131.02 235.53,131.02
S$11652
  Bottom 0: 235.53,131.02 235.6,131.02
S$11653
  Bottom 0: 235.6,131.02 235.67,131.04
S$11654
  Bottom 0: 235.67,131.04 235.73,131.06
S$11655
  Bottom 0: 235.73,131.06 235.79,131.1
S$11656
  Bottom 0: 235.79,131.1 235.84,131.14
S$11657
  Bottom 0: 235.84,131.14 242.61,137.91
S$11658
  Bottom 0: 242.61,137.91 242.65,137.97
S$11659
  Bottom 0: 242.65,137.97 242.7,138.02
S$11660
  Bottom 0: 242.7,138.02 242.72,138.09
S$11661
  Bottom 0: 242.72,138.09 242.74,138.16
S$11662
  Bottom 0: 242.74,138.16 242.74,138.21
S$11663
  Bottom 0: 242.74,138.21 242.81,138.25
S$11664
  Bottom 0: 242.81,138.25 242.94,138.47
S$11665
  Bottom 0: 242.94,138.47 242.99,138.72
S$11666
  Bottom 0: 242.99,138.72 242.94,138.97
S$11667
  Bottom 0: 242.94,138.97 242.94,138.98
S$11668
  Bottom 0: 242.94,138.98 243.15,139.03
S$11669
  Bottom 0: 243.15,139.03 243.2,139.07
S$11670
  Bottom 0: 243.2,139.07 243.2,119.31
S$11671
  Bottom 0: 243.2,119.31 226.34,102.45
S$11672
  Bottom 0: 227.69,104.55 228.01,104.57
S$11673
  Bottom 0: 228.01,104.57 228.32,104.68
S$11674
  Bottom 0: 228.32,104.68 228.58,104.87
S$11675
  Bottom 0: 228.58,104.87 228.79,105.12
S$11676
  Bottom 0: 228.79,105.12 228.91,105.42
S$11677
  Bottom 0: 228.91,105.42 228.96,105.74
S$11678
  Bottom 0: 228.96,105.74 228.91,106.06
S$11679
  Bottom 0: 228.91,106.06 228.79,106.36
S$11680
  Bottom 0: 228.79,106.36 228.58,106.61
S$11681
  Bottom 0: 228.58,106.61 228.34,106.79
S$11682
  Bottom 0: 228.34,106.79 228.34,117.89
S$11683
  Bottom 0: 228.34,117.89 229.57,119.13
S$11684
  Bottom 0: 229.57,119.13 229.82,119.08
S$11685
  Bottom 0: 229.82,119.08 230.15,119.1
S$11686
  Bottom 0: 230.15,119.1 230.45,119.2
S$11687
  Bottom 0: 230.45,119.2 230.72,119.39
S$11688
  Bottom 0: 230.72,119.39 230.93,119.64
S$11689
  Bottom 0: 230.93,119.64 231.05,119.94
S$11690
  Bottom 0: 231.05,119.94 231.1,120.26
S$11691
  Bottom 0: 231.1,120.26 231.05,120.58
S$11692
  Bottom 0: 231.05,120.58 230.93,120.88
S$11693
  Bottom 0: 230.93,120.88 230.72,121.14
S$11694
  Bottom 0: 230.72,121.14 230.45,121.33
S$11695
  Bottom 0: 230.45,121.33 230.15,121.43
S$11696
  Bottom 0: 230.15,121.43 229.82,121.45
S$11697
  Bottom 0: 229.82,121.45 229.57,121.4
S$11698
  Bottom 0: 229.57,121.4 226.53,124.45
S$11699
  Bottom 0: 226.53,124.45 226.53,124.47
S$11700
  Bottom 0: 226.53,124.47 226.58,124.79
S$11701
  Bottom 0: 226.58,124.79 226.53,125.11
S$11702
  Bottom 0: 226.53,125.11 226.4,125.41
S$11703
  Bottom 0: 226.4,125.41 226.2,125.66
S$11704
  Bottom 0: 226.2,125.66 225.93,125.85
S$11705
  Bottom 0: 225.93,125.85 225.63,125.96
S$11706
  Bottom 0: 225.63,125.96 225.3,125.98
S$11707
  Bottom 0: 225.3,125.98 224.98,125.91
S$11708
  Bottom 0: 224.98,125.91 224.69,125.77
S$11709
  Bottom 0: 224.69,125.77 224.46,125.54
S$11710
  Bottom 0: 224.46,125.54 224.29,125.27
S$11711
  Bottom 0: 224.29,125.27 224.2,124.95
S$11712
  Bottom 0: 224.2,124.95 224.2,124.63
S$11713
  Bottom 0: 224.2,124.63 224.29,124.31
S$11714
  Bottom 0: 224.29,124.31 224.46,124.04
S$11715
  Bottom 0: 224.46,124.04 224.69,123.81
S$11716
  Bottom 0: 224.69,123.81 224.98,123.67
S$11717
  Bottom 0: 224.98,123.67 225.3,123.6
S$11718
  Bottom 0: 225.3,123.6 225.63,123.62
S$11719
  Bottom 0: 225.63,123.62 225.72,123.65
S$11720
  Bottom 0: 225.72,123.65 228.77,120.6
S$11721
  Bottom 0: 228.77,120.6 228.72,120.43
S$11722
  Bottom 0: 228.72,120.43 228.72,120.1
S$11723
  Bottom 0: 228.72,120.1 228.77,119.93
S$11724
  Bottom 0: 228.77,119.93 227.37,118.52
S$11725
  Bottom 0: 227.37,118.52 227.31,118.45
S$11726
  Bottom 0: 227.31,118.45 227.26,118.38
S$11727
  Bottom 0: 227.26,118.38 227.22,118.3
S$11728
  Bottom 0: 227.22,118.3 227.2,118.21
S$11729
  Bottom 0: 227.2,118.21 227.2,118.12
S$11730
  Bottom 0: 227.2,118.12 227.2,106.78
S$11731
  Bottom 0: 227.2,106.78 227.08,106.72
S$11732
  Bottom 0: 227.08,106.72 226.84,106.49
S$11733
  Bottom 0: 226.84,106.49 226.67,106.22
S$11734
  Bottom 0: 226.67,106.22 226.58,105.9
S$11735
  Bottom 0: 226.58,105.9 226.58,105.58
S$11736
  Bottom 0: 226.58,105.58 226.67,105.26
S$11737
  Bottom 0: 226.67,105.26 226.84,104.99
S$11738
  Bottom 0: 226.84,104.99 227.08,104.77
S$11739
  Bottom 0: 227.08,104.77 227.37,104.62
S$11740
  Bottom 0: 227.37,104.62 227.69,104.55
S$11741
  Bottom 0: 229.82,111.45 230.15,111.48
S$11742
  Bottom 0: 230.15,111.48 230.45,111.58
S$11743
  Bottom 0: 230.45,111.58 230.72,111.77
S$11744
  Bottom 0: 230.72,111.77 230.93,112.02
S$11745
  Bottom 0: 230.93,112.02 231,112.2
S$11746
  Bottom 0: 231,112.2 232.72,112.2
S$11747
  Bottom 0: 232.72,112.2 232.79,112.21
S$11748
  Bottom 0: 232.79,112.21 232.85,112.22
S$11749
  Bottom 0: 232.85,112.22 232.91,112.25
S$11750
  Bottom 0: 232.91,112.25 232.97,112.29
S$11751
  Bottom 0: 232.97,112.29 233.03,112.33
S$11752
  Bottom 0: 233.03,112.33 241.57,120.87
S$11753
  Bottom 0: 241.57,120.87 241.67,120.86
S$11754
  Bottom 0: 241.67,120.86 241.91,120.92
S$11755
  Bottom 0: 241.91,120.92 242.12,121.08
S$11756
  Bottom 0: 242.12,121.08 242.25,121.29
S$11757
  Bottom 0: 242.25,121.29 242.3,121.54
S$11758
  Bottom 0: 242.3,121.54 242.25,121.79
S$11759
  Bottom 0: 242.25,121.79 242.12,122
S$11760
  Bottom 0: 242.12,122 241.91,122.15
S$11761
  Bottom 0: 241.91,122.15 241.67,122.22
S$11762
  Bottom 0: 241.67,122.22 241.42,122.2
S$11763
  Bottom 0: 241.42,122.2 241.2,122.09
S$11764
  Bottom 0: 241.2,122.09 241.03,121.9
S$11765
  Bottom 0: 241.03,121.9 240.93,121.67
S$11766
  Bottom 0: 240.93,121.67 240.93,121.49
S$11767
  Bottom 0: 240.93,121.49 232.53,113.09
S$11768
  Bottom 0: 232.53,113.09 231,113.09
S$11769
  Bottom 0: 231,113.09 230.93,113.26
S$11770
  Bottom 0: 230.93,113.26 230.72,113.52
S$11771
  Bottom 0: 230.72,113.52 230.45,113.71
S$11772
  Bottom 0: 230.45,113.71 230.15,113.81
S$11773
  Bottom 0: 230.15,113.81 229.82,113.83
S$11774
  Bottom 0: 229.82,113.83 229.5,113.77
S$11775
  Bottom 0: 229.5,113.77 229.22,113.62
S$11776
  Bottom 0: 229.22,113.62 228.98,113.4
S$11777
  Bottom 0: 228.98,113.4 228.81,113.12
S$11778
  Bottom 0: 228.81,113.12 228.72,112.81
S$11779
  Bottom 0: 228.72,112.81 228.72,112.48
S$11780
  Bottom 0: 228.72,112.48 228.81,112.17
S$11781
  Bottom 0: 228.81,112.17 228.98,111.89
S$11782
  Bottom 0: 228.98,111.89 229.22,111.67
S$11783
  Bottom 0: 229.22,111.67 229.5,111.52
S$11784
  Bottom 0: 229.5,111.52 229.82,111.45
S$11785
  Bottom 0: 240.7,130.92 241,130.99
S$11786
  Bottom 0: 241,130.99 241.26,131.14
S$11787
  Bottom 0: 241.26,131.14 241.46,131.36
S$11788
  Bottom 0: 241.46,131.36 241.59,131.63
S$11789
  Bottom 0: 241.59,131.63 241.64,131.93
S$11790
  Bottom 0: 241.64,131.93 241.59,132.23
S$11791
  Bottom 0: 241.59,132.23 241.46,132.51
S$11792
  Bottom 0: 241.46,132.51 241.26,132.72
S$11793
  Bottom 0: 241.26,132.72 241,132.88
S$11794
  Bottom 0: 241,132.88 240.7,132.94
S$11795
  Bottom 0: 240.7,132.94 240.4,132.92
S$11796
  Bottom 0: 240.4,132.92 240.11,132.81
S$11797
  Bottom 0: 240.11,132.81 239.88,132.62
S$11798
  Bottom 0: 239.88,132.62 239.71,132.38
S$11799
  Bottom 0: 239.71,132.38 239.62,132.09
S$11800
  Bottom 0: 239.62,132.09 239.62,131.78
S$11801
  Bottom 0: 239.62,131.78 239.71,131.49
S$11802
  Bottom 0: 239.71,131.49 239.88,131.24
S$11803
  Bottom 0: 239.88,131.24 240.11,131.05
S$11804
  Bottom 0: 240.11,131.05 240.4,130.94
S$11805
  Bottom 0: 240.4,130.94 240.7,130.92
S$11806
  Bottom 0: 209.87,139.45 211.64,139.45
S$11807
  Bottom 0: 211.64,139.45 211.72,139.46
S$11808
  Bottom 0: 211.72,139.46 211.79,139.5
S$11809
  Bottom 0: 211.79,139.5 211.85,139.55
S$11810
  Bottom 0: 211.85,139.55 211.89,139.62
S$11811
  Bottom 0: 211.89,139.62 211.9,139.7
S$11812
  Bottom 0: 211.9,139.7 211.9,141.48
S$11813
  Bottom 0: 211.9,141.48 211.89,141.55
S$11814
  Bottom 0: 211.89,141.55 211.85,141.62
S$11815
  Bottom 0: 211.85,141.62 211.79,141.68
S$11816
  Bottom 0: 211.79,141.68 211.72,141.72
S$11817
  Bottom 0: 211.72,141.72 211.64,141.73
S$11818
  Bottom 0: 211.64,141.73 211.2,141.73
S$11819
  Bottom 0: 211.2,141.73 211.2,141.86
S$11820
  Bottom 0: 211.2,141.86 211.13,142.08
S$11821
  Bottom 0: 211.13,142.08 210.97,142.24
S$11822
  Bottom 0: 210.97,142.24 210.75,142.3
S$11823
  Bottom 0: 210.75,142.3 210.4,142.3
S$11824
  Bottom 0: 210.4,142.3 209.32,143.38
S$11825
  Bottom 0: 209.32,143.38 209.38,143.52
S$11826
  Bottom 0: 209.38,143.52 209.43,143.84
S$11827
  Bottom 0: 209.43,143.84 209.38,144.16
S$11828
  Bottom 0: 209.38,144.16 209.25,144.46
S$11829
  Bottom 0: 209.25,144.46 209.05,144.71
S$11830
  Bottom 0: 209.05,144.71 208.78,144.9
S$11831
  Bottom 0: 208.78,144.9 208.48,145.01
S$11832
  Bottom 0: 208.48,145.01 208.15,145.03
S$11833
  Bottom 0: 208.15,145.03 207.83,144.96
S$11834
  Bottom 0: 207.83,144.96 207.54,144.82
S$11835
  Bottom 0: 207.54,144.82 207.31,144.59
S$11836
  Bottom 0: 207.31,144.59 207.14,144.32
S$11837
  Bottom 0: 207.14,144.32 207.05,144
S$11838
  Bottom 0: 207.05,144 207.05,143.68
S$11839
  Bottom 0: 207.05,143.68 207.14,143.36
S$11840
  Bottom 0: 207.14,143.36 207.31,143.09
S$11841
  Bottom 0: 207.31,143.09 207.54,142.87
S$11842
  Bottom 0: 207.54,142.87 207.83,142.72
S$11843
  Bottom 0: 207.83,142.72 208.15,142.65
S$11844
  Bottom 0: 208.15,142.65 208.48,142.67
S$11845
  Bottom 0: 208.48,142.67 208.7,142.75
S$11846
  Bottom 0: 208.7,142.75 209.75,141.7
S$11847
  Bottom 0: 209.75,141.7 209.72,141.68
S$11848
  Bottom 0: 209.72,141.68 209.66,141.62
S$11849
  Bottom 0: 209.66,141.62 209.62,141.55
S$11850
  Bottom 0: 209.62,141.55 209.61,141.48
S$11851
  Bottom 0: 209.61,141.48 209.61,139.7
S$11852
  Bottom 0: 209.61,139.7 209.62,139.62
S$11853
  Bottom 0: 209.62,139.62 209.66,139.55
S$11854
  Bottom 0: 209.66,139.55 209.72,139.5
S$11855
  Bottom 0: 209.72,139.5 209.79,139.46
S$11856
  Bottom 0: 209.79,139.46 209.87,139.45
S$11857
  Bottom 0: 11.87,103.06 11.85,103.11
S$11858
  Bottom 0: 11.85,103.11 11.64,103.35
S$11859
  Bottom 0: 11.64,103.35 11.36,103.53
S$11860
  Bottom 0: 11.36,103.53 11.05,103.62
S$11861
  Bottom 0: 11.05,103.62 10.73,103.62
S$11862
  Bottom 0: 10.73,103.62 10.42,103.53
S$11863
  Bottom 0: 10.42,103.53 10.14,103.35
S$11864
  Bottom 0: 10.14,103.35 10.05,103.24
S$11865
  Bottom 0: 10.05,103.24 10.05,124.2
S$11866
  Bottom 0: 10.05,124.2 17.57,131.72
S$11867
  Bottom 0: 17.57,131.72 17.59,131.7
S$11868
  Bottom 0: 17.59,131.7 17.93,131.6
S$11869
  Bottom 0: 17.93,131.6 18.27,131.58
S$11870
  Bottom 0: 18.27,131.58 18.62,131.64
S$11871
  Bottom 0: 18.62,131.64 18.94,131.79
S$11872
  Bottom 0: 18.94,131.79 19.21,132.01
S$11873
  Bottom 0: 19.21,132.01 19.37,132.24
S$11874
  Bottom 0: 19.37,132.24 19.37,130.34
S$11875
  Bottom 0: 19.37,130.34 17.34,128.31
S$11876
  Bottom 0: 17.34,128.31 17.24,128.34
S$11877
  Bottom 0: 17.24,128.34 16.92,128.36
S$11878
  Bottom 0: 16.92,128.36 16.6,128.29
S$11879
  Bottom 0: 16.6,128.29 16.31,128.14
S$11880
  Bottom 0: 16.31,128.14 16.08,127.92
S$11881
  Bottom 0: 16.08,127.92 15.9,127.64
S$11882
  Bottom 0: 15.9,127.64 15.82,127.33
S$11883
  Bottom 0: 15.82,127.33 15.82,127
S$11884
  Bottom 0: 15.82,127 15.9,126.69
S$11885
  Bottom 0: 15.9,126.69 16.08,126.42
S$11886
  Bottom 0: 16.08,126.42 16.31,126.19
S$11887
  Bottom 0: 16.31,126.19 16.6,126.05
S$11888
  Bottom 0: 16.6,126.05 16.92,125.98
S$11889
  Bottom 0: 16.92,125.98 17.24,126
S$11890
  Bottom 0: 17.24,126 17.55,126.11
S$11891
  Bottom 0: 17.55,126.11 17.81,126.29
S$11892
  Bottom 0: 17.81,126.29 18.02,126.55
S$11893
  Bottom 0: 18.02,126.55 18.15,126.85
S$11894
  Bottom 0: 18.15,126.85 18.19,127.17
S$11895
  Bottom 0: 18.19,127.17 18.15,127.49
S$11896
  Bottom 0: 18.15,127.49 18.14,127.51
S$11897
  Bottom 0: 18.14,127.51 20.34,129.71
S$11898
  Bottom 0: 20.34,129.71 20.4,129.77
S$11899
  Bottom 0: 20.4,129.77 20.45,129.85
S$11900
  Bottom 0: 20.45,129.85 20.48,129.93
S$11901
  Bottom 0: 20.48,129.93 20.5,130.02
S$11902
  Bottom 0: 20.5,130.02 20.51,130.11
S$11903
  Bottom 0: 20.51,130.11 20.51,135.41
S$11904
  Bottom 0: 20.51,135.41 20.5,135.5
S$11905
  Bottom 0: 20.5,135.5 20.48,135.58
S$11906
  Bottom 0: 20.48,135.58 20.45,135.67
S$11907
  Bottom 0: 20.45,135.67 20.4,135.74
S$11908
  Bottom 0: 20.4,135.74 20.34,135.81
S$11909
  Bottom 0: 20.34,135.81 17.06,139.09
S$11910
  Bottom 0: 17.06,139.09 17.59,139.62
S$11911
  Bottom 0: 17.59,139.62 17.64,139.69
S$11912
  Bottom 0: 17.64,139.69 17.69,139.76
S$11913
  Bottom 0: 17.69,139.76 17.72,139.84
S$11914
  Bottom 0: 17.72,139.84 17.75,139.93
S$11915
  Bottom 0: 17.75,139.93 17.75,140.02
S$11916
  Bottom 0: 17.75,140.02 17.75,142.92
S$11917
  Bottom 0: 17.75,142.92 17.81,142.97
S$11918
  Bottom 0: 17.81,142.97 18.02,143.22
S$11919
  Bottom 0: 18.02,143.22 18.15,143.52
S$11920
  Bottom 0: 18.15,143.52 18.19,143.84
S$11921
  Bottom 0: 18.19,143.84 18.15,144.16
S$11922
  Bottom 0: 18.15,144.16 18.02,144.46
S$11923
  Bottom 0: 18.02,144.46 17.81,144.71
S$11924
  Bottom 0: 17.81,144.71 17.55,144.9
S$11925
  Bottom 0: 17.55,144.9 17.24,145.01
S$11926
  Bottom 0: 17.24,145.01 16.92,145.03
S$11927
  Bottom 0: 16.92,145.03 16.6,144.96
S$11928
  Bottom 0: 16.6,144.96 16.31,144.82
S$11929
  Bottom 0: 16.31,144.82 16.08,144.59
S$11930
  Bottom 0: 16.08,144.59 15.9,144.32
S$11931
  Bottom 0: 15.9,144.32 15.82,144
S$11932
  Bottom 0: 15.82,144 15.82,143.68
S$11933
  Bottom 0: 15.82,143.68 15.9,143.36
S$11934
  Bottom 0: 15.9,143.36 16.08,143.09
S$11935
  Bottom 0: 16.08,143.09 16.31,142.87
S$11936
  Bottom 0: 16.31,142.87 16.6,142.72
S$11937
  Bottom 0: 16.6,142.72 16.62,142.71
S$11938
  Bottom 0: 16.62,142.71 16.62,141.2
S$11939
  Bottom 0: 16.62,141.2 16.61,141.21
S$11940
  Bottom 0: 16.61,141.21 16.4,141.45
S$11941
  Bottom 0: 16.4,141.45 16.12,141.63
S$11942
  Bottom 0: 16.12,141.63 15.81,141.72
S$11943
  Bottom 0: 15.81,141.72 15.49,141.72
S$11944
  Bottom 0: 15.49,141.72 15.18,141.63
S$11945
  Bottom 0: 15.18,141.63 14.9,141.45
S$11946
  Bottom 0: 14.9,141.45 14.69,141.21
S$11947
  Bottom 0: 14.69,141.21 14.55,140.91
S$11948
  Bottom 0: 14.55,140.91 14.51,140.59
S$11949
  Bottom 0: 14.51,140.59 14.55,140.27
S$11950
  Bottom 0: 14.55,140.27 14.69,139.97
S$11951
  Bottom 0: 14.69,139.97 14.9,139.72
S$11952
  Bottom 0: 14.9,139.72 15,139.66
S$11953
  Bottom 0: 15,139.66 14.25,139.66
S$11954
  Bottom 0: 14.25,139.66 14.25,139.7
S$11955
  Bottom 0: 14.25,139.7 14.25,141.48
S$11956
  Bottom 0: 14.25,141.48 14.24,141.55
S$11957
  Bottom 0: 14.24,141.55 14.2,141.62
S$11958
  Bottom 0: 14.2,141.62 14.14,141.68
S$11959
  Bottom 0: 14.14,141.68 14.08,141.72
S$11960
  Bottom 0: 14.08,141.72 14,141.73
S$11961
  Bottom 0: 14,141.73 12.29,141.73
S$11962
  Bottom 0: 12.29,141.73 12.29,150.34
S$11963
  Bottom 0: 12.29,150.34 14.54,152.59
S$11964
  Bottom 0: 14.54,152.59 14.51,152.53
S$11965
  Bottom 0: 14.51,152.53 14.42,152.19
S$11966
  Bottom 0: 14.42,152.19 14.42,151.84
S$11967
  Bottom 0: 14.42,151.84 14.51,151.51
S$11968
  Bottom 0: 14.51,151.51 14.68,151.2
S$11969
  Bottom 0: 14.68,151.2 14.92,150.94
S$11970
  Bottom 0: 14.92,150.94 15.21,150.75
S$11971
  Bottom 0: 15.21,150.75 15.54,150.65
S$11972
  Bottom 0: 15.54,150.65 15.89,150.63
S$11973
  Bottom 0: 15.89,150.63 16.24,150.69
S$11974
  Bottom 0: 16.24,150.69 16.56,150.84
S$11975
